(* Logix 5000 AddOnInstructionDefinition export ACS_FAULTS_CRITICAL_ACTIVE; software revision 20.01 *)

TYPE DriveFaults :
STRUCT
   Positive_Limit : BOOL;   // Positive Limit
   Negative_Limit : BOOL;   // Negative Limit
   E_Stop : BOOL;   // E Stop
   Position_Error : BOOL;   // Position Error
   Feedback_Error : BOOL;   // Feedback Error
   Over_Current : BOOL;   // Overcurrent
   Motor_Over_Temperature : BOOL;   // Motor Over Temperature
   Drive_Over_Temperature : BOOL;   // Drive Over Temperature
   Drive_Over_Voltage : BOOL;   // Drive Over Voltage
   Drive_Under_Voltage : BOOL;   // Drive Under Voltage
   Flash_Error : BOOL;   // Flash Error
   I2T_Limit : BOOL;   // I2T Limit Fault
   Short_Circuit : BOOL;   // Short Circuit Fault
   Watchdog_Reset : BOOL;   // Watchdog Reset
END_STRUCT
END_TYPE

ADD_ON_INSTRUCTION ACS_FAULTS_CRITICAL_ACTIVE   (* revision 2.0, vendor Tolomatic, Inc *)
// Determines if ACS drive has any Critical Faults active
VAR_IN_OUT
   DriveFaults : DINT; {required}   // ACS.I.FAULTS
END_VAR
VAR
   LocalFaults : DriveFaults; {access None}   // Local Storage for decoding faults
END_VAR

ROUTINE Logic   (* ladder *)
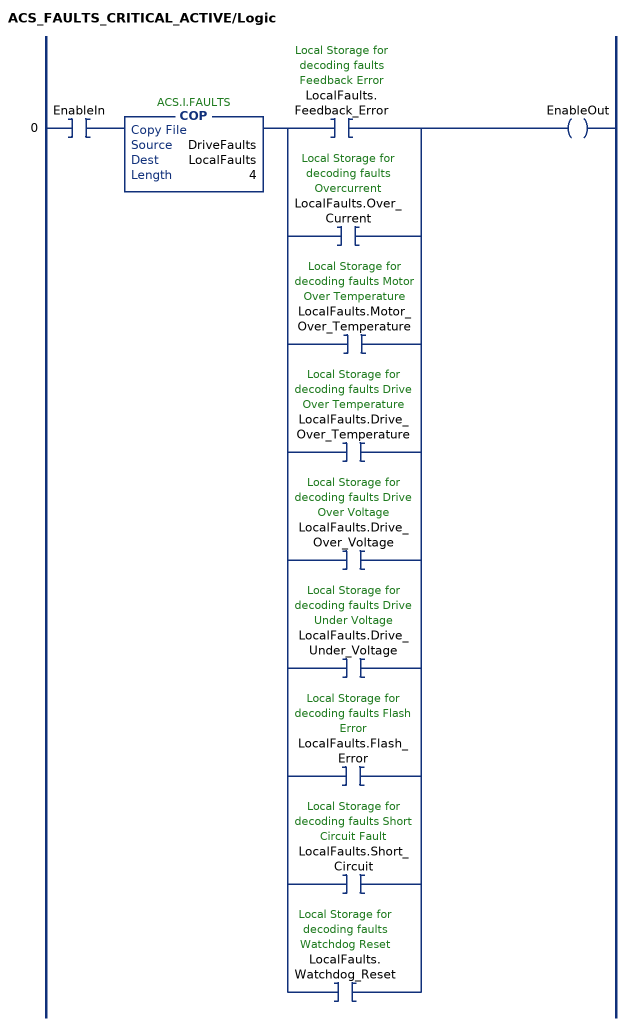
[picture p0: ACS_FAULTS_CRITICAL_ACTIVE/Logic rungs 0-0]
   0: XIC(EnableIn)COP(DriveFaults,LocalFaults,4)[XIC(LocalFaults.Feedback_Error) ,XIC(LocalFaults.Over_Current) ,XIC(LocalFaults.Motor_Over_Temperature) ,XIC(LocalFaults.Drive_Over_Temperature) ,XIC(LocalFaults.Drive_Over_Voltage) ,XIC(LocalFaults.Drive_Under_Voltage) ,XIC(LocalFaults.Flash_Error) ,XIC(LocalFaults.Short_Circuit) ,XIC(LocalFaults.Watchdog_Reset) ]OTE(EnableOut);
END_ROUTINE
END_ADD_ON_INSTRUCTION
